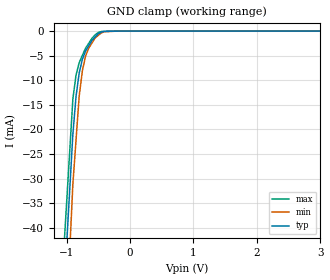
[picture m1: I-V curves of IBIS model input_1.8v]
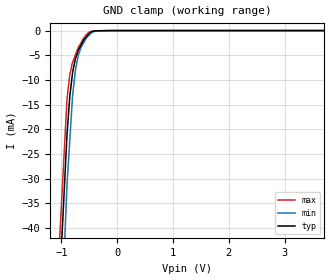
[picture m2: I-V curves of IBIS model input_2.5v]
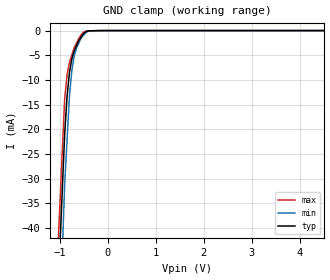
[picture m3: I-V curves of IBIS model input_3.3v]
| Teraspeed Modeling Services.
| http://www.teraspeed.com
[IBIS Ver]   4.0
[Comment Char] |_char
[File Name]   lpc810m021fn8.ibs
[File Rev]   3.0
[Source]  Measured and created by Teraspeed Consulting Group LLC
[Date]   08-09-2013
[Notes]   Quality Check of this IBIS model: Model Passes IBIS Check
   Model parses into ICX IS. Simulation done with Hyperlynx.
   1. MIN TYP MAX information is based on Temperature and Voltage
   characteristics only.
   2. Package data measured using Tektronix IConnect Software.
   3. This model standard temperature range:  -40 to +85
[Disclaimer]
| Use: Teraspeed Consulting Group LLC ("Teraspeed") has
| licensed IBIS models to specific integrated circuit
| suppliers ("IC Vendors") for use and distribustion as
| follows: Each IC Vendor may use IBIS Models, and distribute
| them to IC Vendor's custumers to use solely for developing
| printed circute board designs. Users of this model may
| modify the IBIS model to suit its specific applications but
| rights to derivative works and such modifications shall belong
| to Teraspeed. No other distribution of these materials is
| permitted.
| DISCLAIMER OF WARRANTY: UNLESS OTHERWISE AGREED TO IN WRITING
| TERASPEED DISCLAIMS AND USER WAIVES ALL WARRANTIES, EXPRESS
| OR IMPLIED, INCLUDING WARRANTIES OF MERCHANTABILITY AND
| FITNESS FOR A PARTICULAR PURPOSE. IN NO EVENT SHALL
| TERASPEED BE LIABLE FOR ANY DIRECT OR INDIRECT DAMAGES,
| WHETHER IN CONTRACT OR TORT, INCLUDING, WITHOUT LIMITATION,
| LOST PROFITS, BUSINESS INTERRUPTION, OR LOST INFORMATION
| ARISING OUT OF THE USE OF OR THE INABILITY TO USE THE MODEL,
| EVEN IF TERASPEED HAS BEEN ADVISED OF THE POSSIBILITY OF SUCH
| DAMAGES.
[Copyright]
| This file is the legal property of Teraspeed Copyright(c) 2013.
| All other rights are reserved.
[Component] LPC810M021FN8
[Manufacturer] NXP Semiconductors
[Package]
| DIP8/SOT97-2
| variable   typ   min   max
R_pkg  1.000E-02  1.000E-02  1.000E-02
L_pkg  2.825E-09  2.610E-09  3.040E-09
C_pkg  5.090E-13  4.660E-13  5.520E-13
[Pin] signal_name  model_name  R_pin  L_pin C_pin
1   *RESET/PIO0_5   pio0_5   1.000E-02   3.040E-09   5.520E-13
2   PIO0_4/WAKEUP/*TRST   pio0_4   1.000E-02   2.610E-09   4.660E-13
3   SWCLK/PIO0_3/TCK   pio0_3   1.000E-02   2.610E-09   4.660E-13
4   SWDIO/PIO0_2/TMS   pio0_2   1.000E-02   3.040E-09   5.520E-13
5   PIO0_1/CMPI2/CLK/TDI   pio0_1   1.000E-02   3.040E-09   5.520E-13
6   VDD   POWER   1.000E-02   2.610E-09   4.660E-13
7   VSS   GND   1.000E-02   2.610E-09   4.660E-13
8   PIO0_0/CMPI1/TDO   pio0_0   1.000E-02   3.040E-09   5.520E-13
|******Normal Drive I/O's******
[Model Selector]  pio0_4
input_1.8v   input,no int pd/pu,vdd=1.8v
input_2.5v   input,no int pd/pu,vdd=2.5v
input_3.3v   input,no int pd/pu,vdd=3.3v
pd_1.8v   input,int pd,vdd=1.8v
pd_2.5v   input,int pd,vdd=2.5v
pd_3.3v   input,int pd,vdd=3.3v
pu_1.8v   input,int pu,vdd=1.8v | PWR-UP Default
pu_2.5v   input,int pu,vdd=2.5v | PWR-UP Default
pu_3.3v   input,int pu,vdd=3.3v | PWR-UP Default
io_1.8v   io,vdd=1.8v
io_2.5v   io,vdd=2.5v
io_3.3v   io,vdd=3.3v
io_odf_1.8v   fast open drain io,vdd=1.8v
io_odf_2.5v   fast open drain io,vdd=2.5v
io_odf_3.3v   fast open drain io,vdd=3.3v
[Model Selector]  pio0_5
input_1.8v   input,no int pd/pu,vdd=1.8v
input_2.5v   input,no int pd/pu,vdd=2.5v
input_3.3v   input,no int pd/pu,vdd=3.3v
pd_1.8v   input,int pd,vdd=1.8v
pd_2.5v   input,int pd,vdd=2.5v
pd_3.3v   input,int pd,vdd=3.3v
pu_1.8v   input,int pu,vdd=1.8v | PWR-UP/Reset Default
pu_2.5v   input,int pu,vdd=2.5v | PWR-UP/Reset Default
pu_3.3v   input,int pu,vdd=3.3v | PWR-UP/Reset Default
io_1.8v   io,vdd=1.8v
io_2.5v   io,vdd=2.5v
io_3.3v   io,vdd=3.3v
io_odf_1.8v   fast open drain io,vdd=1.8v
io_odf_2.5v   fast open drain io,vdd=2.5v
io_odf_3.3v   fast open drain io,vdd=3.3v
|******Normal Drive I/O's w/Analog Func ******
[Model Selector]  pio0_0
input_1.8v   input,no int pd/pu,vdd=1.8v
input_2.5v   input,no int pd/pu,vdd=2.5v
input_3.3v   input,no int pd/pu,vdd=3.3v
pd_1.8v   input,int pd,vdd=1.8v
pd_2.5v   input,int pd,vdd=2.5v
pd_3.3v   input,int pd,vdd=3.3v
pu_1.8v   input,int pu,vdd=1.8v | PWR-UP/Reset Default
pu_2.5v   input,int pu,vdd=2.5v | PWR-UP/Reset Default
pu_3.3v   input,int pu,vdd=3.3v | PWR-UP/Reset Default
io_1.8v   io,vdd=1.8v
io_2.5v   io,vdd=2.5v
io_3.3v   io,vdd=3.3v
io_odf_1.8v   fast open drain io,vdd=1.8v
io_odf_2.5v   fast open drain io,vdd=2.5v
io_odf_3.3v   fast open drain io,vdd=3.3v
term   analog comparator input1
[Model Selector]  pio0_1
input_1.8v   input,no int pd/pu,vdd=1.8v
input_2.5v   input,no int pd/pu,vdd=2.5v
input_3.3v   input,no int pd/pu,vdd=3.3v
pd_1.8v   input,int pd,vdd=1.8v
pd_2.5v   input,int pd,vdd=2.5v
pd_3.3v   input,int pd,vdd=3.3v
pu_1.8v   input,int pu,vdd=1.8v | PWR-UP/Reset Default
pu_2.5v   input,int pu,vdd=2.5v | PWR-UP/Reset Default
pu_3.3v   input,int pu,vdd=3.3v | PWR-UP/Reset Default
io_1.8v   io,vdd=1.8v
io_2.5v   io,vdd=2.5v
io_3.3v   io,vdd=3.3v
io_odf_1.8v   fast open drain io,vdd=1.8v
io_odf_2.5v   fast open drain io,vdd=2.5v
io_odf_3.3v   fast open drain io,vdd=3.3v
term   analog comparator input2
|******High Drive(source) I/O's******
[Model Selector]  pio0_2
input_1.8v   input,no int pd/pu,vdd=1.8v
input_2.5v   input,no int pd/pu,vdd=2.5v
input_3.3v   input,no int pd/pu,vdd=3.3v
pd_1.8v   input,int pd,vdd=1.8v
pd_2.5v   input,int pd,vdd=2.5v
pd_3.3v   input,int pd,vdd=3.3v
pu_1.8v   input,int pu,vdd=1.8v | PWR-UP/Reset Default
pu_2.5v   input,int pu,vdd=2.5v | PWR-UP/Reset Default
pu_3.3v   input,int pu,vdd=3.3v | PWR-UP/Reset Default
hi_drv_io_1.8v  io,hi src drv,vdd=1.8v
hi_drv_io_2.5v  io,hi src drv,vdd=2.5v
hi_drv_io_3.3v  io,hi src drv,vdd=3.3v
io_ods_1.8v   slow open drain io,vdd=1.8v
io_ods_2.5v   slow open drain io,vdd=2.5v
io_ods_3.3v   slow open drain io,vdd=3.3v
[Model Selector]  pio0_3
input_1.8v   input,no int pd/pu,vdd=1.8v
input_2.5v   input,no int pd/pu,vdd=2.5v
input_3.3v   input,no int pd/pu,vdd=3.3v
pd_1.8v   input,int pd,vdd=1.8v
pd_2.5v   input,int pd,vdd=2.5v
pd_3.3v   input,int pd,vdd=3.3v
pu_1.8v   input,int pu,vdd=1.8v | PWR-UP/Reset Default
pu_2.5v   input,int pu,vdd=2.5v | PWR-UP/Reset Default
pu_3.3v   input,int pu,vdd=3.3v | PWR-UP/Reset Default
hi_drv_io_1.8v  io,hi src drv,vdd=1.8v
hi_drv_io_2.5v  io,hi src drv,vdd=2.5v
hi_drv_io_3.3v  io,hi src drv,vdd=3.3v
io_ods_1.8v   slow open drain io,vdd=1.8v
io_ods_2.5v   slow open drain io,vdd=2.5v
io_ods_3.3v   slow open drain io,vdd=3.3v
[Model] term
Model_type Terminator
C_comp  0pF 0pF 0pF
| variable typ   min   max
[Voltage Range]   3.30000V  3.00000V  3.60000V
[POWER Clamp Reference]  3.30000V  3.00000V  3.60000V
[GND Clamp Reference]   0.00000V  0.00000V  0.00000V
[Temperature Range]   25   85   -40
| Models and submodels in the file (22): input_1.8v (Input), input_2.5v (Input), input_3.3v (Input), pd_1.8v (Input), pd_2.5v (Input), pd_3.3v (Input), pu_1.8v (Input), pu_2.5v (Input), pu_3.3v (Input), hi_drv_io_1.8v (I/O), hi_drv_io_2.5v (I/O), hi_drv_io_3.3v (I/O), io_1.8v (I/O), io_2.5v (I/O), io_3.3v (I/O), io_odf_1.8v (I/O_open_drain), io_odf_2.5v (I/O_open_drain), io_odf_3.3v (I/O_open_drain), io_ods_1.8v (I/O_open_drain), io_ods_2.5v (I/O_open_drain), io_ods_3.3v (I/O_open_drain), term (Terminator)
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[Model] input_1.8v
Model_type Input
Vinl = 540.000mV
Vinh = 1.26000V
C_comp 909.000fF 904.000fF 914.000fF
| variable typ   min   max
[Voltage Range] 1.80000V 1.65000V 1.95000V
[POWER Clamp Reference] 1.80000V 1.65000V 1.95000V
[GND Clamp Reference] 0.00000V 0.00000V 0.00000V
[Temperature Range]   25   85   -40
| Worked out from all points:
|   GND clamp passes 1 mA (typ) near -0.53 V on its own axis
[GND Clamp]
-1.8V     -226.1mA   -279.2mA   -207.1mA
-900mV    -20.98mA   -31.13mA   -13.8mA
-850mV    -13.28mA   -22.15mA   -8.911mA
-800mV    -8.483mA   -13.16mA   -6.412mA
-750mV    -5.729mA   -8.059mA   -4.946mA
-700mV    -4.056mA   -5.078mA   -3.479mA
-650mV    -2.988mA   -3.465mA   -2.487mA
-550mV    -1.226mA   -1.411mA   -758.6uA
-500mV    -532.9uA   -883.1uA   -295.9uA
-400mV    -46.91uA   -121.5uA   -71.69uA
-200mV    -8.97uA    -6.932uA   -21.03uA
3.6V      0A         0A         0A
[POWER Clamp]
-1.8V     0A         0A         0A
3.6V      0A         0A         0A
[Model] input_2.5v
Model_type Input
Vinl = 750.000mV
Vinh = 1.75000V
C_comp 587.000fF 585.000fF 589.000fF
| variable typ   min   max
[Voltage Range] 2.50000V 2.25000V 2.75000V
[POWER Clamp Reference] 2.50000V 2.25000V 2.75000V
[GND Clamp Reference] 0.00000V 0.00000V 0.00000V
[Temperature Range]   25   85   -40
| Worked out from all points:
|   GND clamp passes 1 mA (typ) near -0.53 V on its own axis
[GND Clamp]
-2.5V     -385.6mA   -472.2mA   -357.5mA
-900mV    -20.98mA   -31.13mA   -13.8mA
-850mV    -13.28mA   -22.15mA   -8.911mA
-800mV    -8.483mA   -13.16mA   -6.412mA
-750mV    -5.729mA   -8.059mA   -4.946mA
-700mV    -4.056mA   -5.078mA   -3.479mA
-650mV    -2.988mA   -3.465mA   -2.487mA
-550mV    -1.226mA   -1.411mA   -758.6uA
-500mV    -532.9uA   -883.1uA   -295.9uA
-400mV    -46.91uA   -121.5uA   -71.69uA
-200mV    -8.97uA    -6.932uA   -21.03uA
5V        0A         0A         0A
[POWER Clamp]
-2.5V     0A         0A         0A
5V        0A         0A         0A
[Model] input_3.3v
Model_type Input
Vinl = 990.000mV
Vinh = 2.31000V
C_comp 587.000fF 585.000fF 589.000fF
| variable typ   min   max
[Voltage Range] 3.30000V 3.00000V 3.60000V
[POWER Clamp Reference] 3.30000V 3.00000V 3.60000V
[GND Clamp Reference] 0.00000V 0.00000V 0.00000V
[Temperature Range]   25   85   -40
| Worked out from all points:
|   GND clamp passes 1 mA (typ) near -0.53 V on its own axis
[GND Clamp]
-3.3V     -567.9mA   -692.8mA   -529.3mA
-900mV    -20.98mA   -31.13mA   -13.8mA
-850mV    -13.28mA   -22.15mA   -8.911mA
-800mV    -8.483mA   -13.16mA   -6.412mA
-750mV    -5.729mA   -8.059mA   -4.946mA
-700mV    -4.056mA   -5.078mA   -3.479mA
-650mV    -2.988mA   -3.465mA   -2.487mA
-600mV    -1.919mA   -2.438mA   -1.496mA
-550mV    -1.226mA   -1.411mA   -758.6uA
-450mV    -189.9uA   -355.1uA   -86.11uA
-200mV    -8.97uA    -6.932uA   -21.03uA
6.6V      0A         0A         0A
[POWER Clamp]
-3.3V     0A         0A         0A
6.6V      0A         0A         0A
